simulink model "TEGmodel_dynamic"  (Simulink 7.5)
settings: Solver=ode23s  StartTime=0.0  StopTime=0.01  RelTol=1e-3
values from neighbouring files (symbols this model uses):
  alpha = 0.000382    [TEGmodel_contactR.m]    (also in TEGmodel_parameters.m; TEGmodel_simplified.m)
  mtcs = 0.4492*7.7/1000    (= 0.00345884)    [TEGmodel_parameters.m]
  N = 72    [TEGmodel_contactR.m]    (also in TEGmodel_parameters.m; TEGmodel_simplified.m)
  Ri = 10.2    [TEGmodel_parameters.m]    (also in TEGmodel_simplified.m)
  RL = 10.2    [TEGmodel_parameters.m]    (also in TEGmodel_simplified.m)
  TC = 35 + CtoK    (= 308.15)    [TEGmodel_contactR.m]    (also in TEGmodel_parameters.m; TEGmodel_simplified.m = 35)
  TH = 85 + CtoK    (= 358.15)    [TEGmodel_contactR.m]    (also in TEGmodel_parameters.m; TEGmodel_simplified.m = 85)
libraries: fl_lib x30, nesl_utility x13

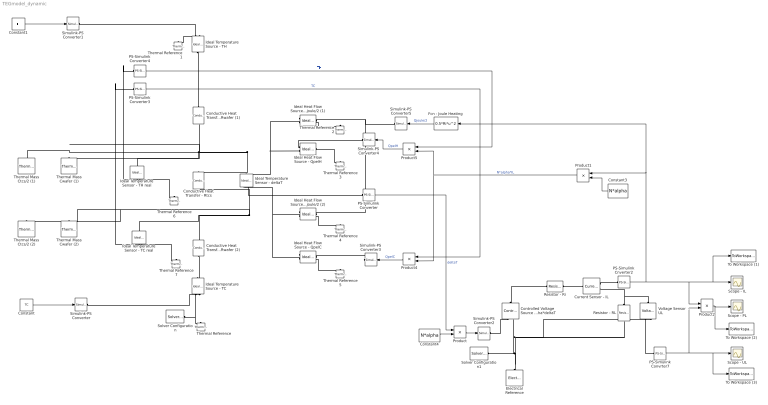
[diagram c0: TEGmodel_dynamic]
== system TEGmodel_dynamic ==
  Conductive Heat Transfer - Rtcs : fl_lib/Thermal/Thermal Elements/Conductive Heat Transfer  DialogController=NetworkEngine.DynNeDlgSource  SystemSampleTime=-1  area=Atcs mm^2  thickness=ttcs mm  th_cond=ktcs W/(m*K)  Q_Log=off  T_Log=off  LocalVarNames=|Q|T  LocalVarDescs=|Q|T  LocalVarLogging=[0 0]
  Conductive Heat Transfer - Rwafer (1) : fl_lib/Thermal/Thermal Elements/Conductive Heat Transfer  DialogController=NetworkEngine.DynNeDlgSource  SystemSampleTime=-1  area=Awafer mm^2  thickness=twafer mm  th_cond=kwafer W/(m*K)  Q_Log=off  T_Log=off  LocalVarNames=|Q|T  LocalVarDescs=|Q|T  LocalVarLogging=[0 0]
  Conductive Heat Transfer - Rwafer (2) : fl_lib/Thermal/Thermal Elements/Conductive Heat Transfer  DialogController=NetworkEngine.DynNeDlgSource  SystemSampleTime=-1  area=Awafer mm^2  thickness=twafer mm  th_cond=kwafer W/(m*K)  Q_Log=off  T_Log=off  LocalVarNames=|Q|T  LocalVarDescs=|Q|T  LocalVarLogging=[0 0]
  Constant : Constant  Value=TC  OutDataType=fixdt(1, 16)  OutScaling=2^0
  Constant1 : Constant  Value=TH  OutDataType=fixdt(1, 16)  OutScaling=2^0
  Constant3 : Constant  Value=N*alpha  OutDataType=fixdt(1, 16)  OutScaling=2^0
  Constant4 : Constant  Value=N*alpha  OutDataType=fixdt(1, 16)  OutScaling=2^0
  Controlled Voltage Source  - N*alpha*deltaT : fl_lib/Electrical/Electrical Sources/Controlled Voltage Source  DialogController=NetworkEngine.DynNeDlgSource  SystemSampleTime=-1  i_Log=off  v_Log=off  LocalVarNames=|i|v  LocalVarDescs=|i|v  LocalVarLogging=[0 0]
  Current Sensor - IL : fl_lib/Electrical/Electrical Sensors/Current Sensor  DialogController=NetworkEngine.DynNeDlgSource  SystemSampleTime=-1  i1_Log=off  v1_Log=off  LocalVarNames=|i1|v1  LocalVarDescs=|i1|v1  LocalVarLogging=[0 0]
  Electrical Reference : fl_lib/Electrical/Electrical Elements/Electrical Reference  DialogController=NetworkEngine.DynNeDlgSource  SystemSampleTime=-1  i_Log=off  LocalVarNames=|i  LocalVarDescs=|i  LocalVarLogging=0
  Fcn - Joule Heating : Fcn  Expr=0.5*Ri*u^2
  Ideal Heat Flow Source - Qjoule/2 (1) : fl_lib/Thermal/Thermal Sources/Ideal Heat Flow Source  DialogController=NetworkEngine.DynNeDlgSource  SystemSampleTime=-1  Q_Log=off  T_Log=off  LocalVarNames=|Q|T  LocalVarDescs=|Q|T  LocalVarLogging=[0 0]
  Ideal Heat Flow Source - Qjoule/2 (2) : fl_lib/Thermal/Thermal Sources/Ideal Heat Flow Source  DialogController=NetworkEngine.DynNeDlgSource  SystemSampleTime=-1  Q_Log=off  T_Log=off  LocalVarNames=|Q|T  LocalVarDescs=|Q|T  LocalVarLogging=[0 0]
  Ideal Heat Flow Source - QpelC : fl_lib/Thermal/Thermal Sources/Ideal Heat Flow Source  DialogController=NetworkEngine.DynNeDlgSource  SystemSampleTime=-1  Q_Log=off  T_Log=off  LocalVarNames=|Q|T  LocalVarDescs=|Q|T  LocalVarLogging=[0 0]
  Ideal Heat Flow Source - QpelH : fl_lib/Thermal/Thermal Sources/Ideal Heat Flow Source  DialogController=NetworkEngine.DynNeDlgSource  SystemSampleTime=-1  Q_Log=off  T_Log=off  LocalVarNames=|Q|T  LocalVarDescs=|Q|T  LocalVarLogging=[0 0]
  Ideal Temperature Sensor - TC real : fl_lib/Thermal/Thermal Sensors/Ideal Temperature Sensor  DialogController=NetworkEngine.DynNeDlgSource  SystemSampleTime=-1  Qs_Log=off  Ts_Log=off  LocalVarNames=|Qs|Ts  LocalVarDescs=|Qs|Ts  LocalVarLogging=[0 0]
  Ideal Temperature Sensor - TH real : fl_lib/Thermal/Thermal Sensors/Ideal Temperature Sensor  DialogController=NetworkEngine.DynNeDlgSource  SystemSampleTime=-1  Qs_Log=off  Ts_Log=off  LocalVarNames=|Qs|Ts  LocalVarDescs=|Qs|Ts  LocalVarLogging=[0 0]
  Ideal Temperature Sensor - deltaT : fl_lib/Thermal/Thermal Sensors/Ideal Temperature Sensor  DialogController=NetworkEngine.DynNeDlgSource  SystemSampleTime=-1  Qs_Log=off  Ts_Log=off  LocalVarNames=|Qs|Ts  LocalVarDescs=|Qs|Ts  LocalVarLogging=[0 0]
  Ideal Temperature Source - TC : fl_lib/Thermal/Thermal Sources/Ideal Temperature Source  DialogController=NetworkEngine.DynNeDlgSource  SystemSampleTime=-1  Q_Log=off  T_Log=off  LocalVarNames=|Q|T  LocalVarDescs=|Q|T  LocalVarLogging=[0 0]
  Ideal Temperature Source - TH : fl_lib/Thermal/Thermal Sources/Ideal Temperature Source  DialogController=NetworkEngine.DynNeDlgSource  SystemSampleTime=-1  Q_Log=off  T_Log=off  LocalVarNames=|Q|T  LocalVarDescs=|Q|T  LocalVarLogging=[0 0]
  PS-Simulink Cnverter2 : nesl_utility/PS-Simulink Converter  DialogController=NetworkEngine.DynNeUtilDlgSource  SystemSampleTime=-1  PhysicalDomain=network_engine_domain  LeftPortType=input  RightPortType=output  SubClassName=ps_output  Unit=1  AffineConversion=off
  PS-Simulink Converter : nesl_utility/PS-Simulink Converter  DialogController=NetworkEngine.DynNeUtilDlgSource  SystemSampleTime=-1  PhysicalDomain=network_engine_domain  LeftPortType=input  RightPortType=output  SubClassName=ps_output  Unit=1  AffineConversion=off
  PS-Simulink Converter3 : nesl_utility/PS-Simulink Converter  DialogController=NetworkEngine.DynNeUtilDlgSource  SystemSampleTime=-1  PhysicalDomain=network_engine_domain  LeftPortType=input  RightPortType=output  SubClassName=ps_output  Unit=1  AffineConversion=off
  PS-Simulink Converter4 : nesl_utility/PS-Simulink Converter  DialogController=NetworkEngine.DynNeUtilDlgSource  SystemSampleTime=-1  PhysicalDomain=network_engine_domain  LeftPortType=input  RightPortType=output  SubClassName=ps_output  Unit=1  AffineConversion=off
  PS-Simulink Convrter7 : nesl_utility/PS-Simulink Converter  DialogController=NetworkEngine.DynNeUtilDlgSource  SystemSampleTime=-1  PhysicalDomain=network_engine_domain  LeftPortType=input  RightPortType=output  SubClassName=ps_output  Unit=1  AffineConversion=off
  Product{,1..2,4..5} (5 alike) : Product  OutDataType=fixdt(1, 16)  OutScaling=2^0
  Resistor - RL : fl_lib/Electrical/Electrical Elements/Resistor  DialogController=NetworkEngine.DynNeDlgSource  SystemSampleTime=-1  R=RL Ohm  i_Log=off  v_Log=off  LocalVarNames=|i|v  LocalVarDescs=|i|v  LocalVarLogging=[0 0]
  Resistor - Ri : fl_lib/Electrical/Electrical Elements/Resistor  DialogController=NetworkEngine.DynNeDlgSource  SystemSampleTime=-1  R=Ri Ohm  i_Log=off  v_Log=off  LocalVarNames=|i|v  LocalVarDescs=|i|v  LocalVarLogging=[0 0]
  Scope - IL : Scope
  Scope - PL : Scope
  Scope - UL : Scope
  Simulink-PS Converter{,1..5} (6 alike) : nesl_utility/Simulink-PS Converter  DialogController=NetworkEngine.DynNeUtilDlgSource  SystemSampleTime=-1  PhysicalDomain=network_engine_domain  LeftPortType=input  RightPortType=output  SubClassName=ps_input  Unit=1  AffineConversion=off  InputFilterTimeConstant=.001  UdotUserProvided=0
  Solver Configuration : nesl_utility/Solver Configuration  DialogController=NetworkEngine.DynNeUtilDlgSource  SystemSampleTime=-1  PhysicalDomain=network_engine_domain  LeftPortType=input  RightPortType=generic  SubClassName=solver  Accelerate=off  Profile=off  ResidualTolerance=1e-9  MaxNonlinIter=3  MaxModeIter=2  DoFixedCost=off  UseLocalSampling=off  DoDC=off  LinearAlgebra=Sparse  LocalSolverSampleTime=.001  LocalSolverChoice=NE_BACKWARD_EULER_ADVANCER  UseLocalSolver=off
  Solver Configuration1 : nesl_utility/Solver Configuration  DialogController=NetworkEngine.DynNeUtilDlgSource  SystemSampleTime=-1  PhysicalDomain=network_engine_domain  LeftPortType=input  RightPortType=generic  SubClassName=solver  Accelerate=off  Profile=off  ResidualTolerance=1e-9  MaxNonlinIter=3  MaxModeIter=2  DoFixedCost=off  UseLocalSampling=off  DoDC=off  LinearAlgebra=Sparse  LocalSolverSampleTime=.001  LocalSolverChoice=NE_BACKWARD_EULER_ADVANCER  UseLocalSolver=off
  Thermal Mass Ctcs/2 (1) : fl_lib/Thermal/Thermal Elements/Thermal Mass  DialogController=NetworkEngine.DynNeDlgSource  SystemSampleTime=-1  mass=mtcs/2 g  sp_heat=Cspecwafer J/kg/K  init_temp=TC K  Q_Log=off  LocalVarNames=|Q  LocalVarDescs=|Q  LocalVarLogging=0
  Thermal Mass Ctcs/2 (2) : fl_lib/Thermal/Thermal Elements/Thermal Mass  DialogController=NetworkEngine.DynNeDlgSource  SystemSampleTime=-1  mass=mtcs/2 g  sp_heat=Cspectcs J/kg/K  init_temp=TC K  Q_Log=off  LocalVarNames=|Q  LocalVarDescs=|Q  LocalVarLogging=0
  Thermal Mass Cwafer (1) : fl_lib/Thermal/Thermal Elements/Thermal Mass  DialogController=NetworkEngine.DynNeDlgSource  SystemSampleTime=-1  mass=mwafer g  sp_heat=Cspecwafer J/kg/K  init_temp=TC K  Q_Log=off  LocalVarNames=|Q  LocalVarDescs=|Q  LocalVarLogging=0
  Thermal Mass Cwafer (2) : fl_lib/Thermal/Thermal Elements/Thermal Mass  DialogController=NetworkEngine.DynNeDlgSource  SystemSampleTime=-1  mass=mwafer g  sp_heat=Cspecwafer J/kg/K  init_temp=TC K  Q_Log=off  LocalVarNames=|Q  LocalVarDescs=|Q  LocalVarLogging=0
  Thermal Reference{,1..7} (8 alike) : fl_lib/Thermal/Thermal Elements/Thermal Reference  DialogController=NetworkEngine.DynNeDlgSource  SystemSampleTime=-1  Q_Log=off  LocalVarNames=|Q  LocalVarDescs=|Q  LocalVarLogging=0
  To Workspace (1) : ToWorkspace  VariableName=IL  SampleTime=-1  SaveFormat=Array
  To Workspace (2) : ToWorkspace  VariableName=PL  SampleTime=-1  SaveFormat=Array
  To Workspace (3) : ToWorkspace  VariableName=UL  SampleTime=-1  SaveFormat=Array
  Voltage Sensor  - UL : fl_lib/Electrical/Electrical Sensors/Voltage Sensor  DialogController=NetworkEngine.DynNeDlgSource  SystemSampleTime=-1  i1_Log=off  v1_Log=off  LocalVarNames=|i1|v1  LocalVarDescs=|i1|v1  LocalVarLogging=[0 0]
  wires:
  Constant/1 -> Simulink-PS Converter/1
  Constant1/1 -> Simulink-PS Converter1/1
  Product/1 -> Simulink-PS Converter2/1
  PS-Simulink Cnverter2/1 -> Product2/1, Scope - IL/1, To Workspace (1)/1, Fcn - Joule Heating/1, Product1/1
  PS-Simulink Convrter7/1 -> Product2/2, Scope - UL/1, To Workspace (3)/1
  Fcn - Joule Heating/1 -> Simulink-PS Converter5/1  "Qjoule/2"
  PS-Simulink Converter/1 -> Product/1  "deltaT"
  Constant4/1 -> Product/2
  PS-Simulink Converter3/1 -> Product4/1  "TC"
  Product4/1 -> Simulink-PS Converter3/1  "QpelC"
  Product5/1 -> Simulink-PS Converter4/1  "QpelH"
  PS-Simulink Converter4/1 -> Product5/1  "TH"
  Product2/1 -> Scope - PL/1, To Workspace (2)/1
  Product1/1 -> Product5/2, Product4/2  "N*alpha*IL"
  Constant3/1 -> Product1/2
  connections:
  Solver Configuration/RConn1 -- Thermal Reference/LConn1 -- Ideal Temperature Source - TC/RConn2
  Ideal Heat Flow Source - Qjoule/2 (1)/LConn1 -- Conductive Heat Transfer - Rtcs/RConn1 -- Ideal Temperature Sensor - TH real/LConn1 -- Conductive Heat Transfer - Rwafer (1)/LConn1 -- Thermal Mass Ctcs/2 (1)/LConn1 -- Thermal Mass Cwafer (1)/LConn1 -- Ideal Heat Flow Source - QpelH/RConn2 -- Ideal Temperature Sensor - deltaT/LConn1
  Ideal Heat Flow Source - QpelH/LConn1 -- Thermal Reference3/LConn1
  Ideal Heat Flow Source - Qjoule/2 (1)/RConn2 -- Thermal Reference2/LConn1
  Ideal Heat Flow Source - Qjoule/2 (2)/RConn2 -- Thermal Reference4/LConn1
  Ideal Heat Flow Source - QpelC/RConn2 -- Thermal Reference5/LConn1
  Ideal Heat Flow Source - QpelC/LConn1 -- Ideal Heat Flow Source - Qjoule/2 (2)/LConn1 -- Conductive Heat Transfer - Rtcs/LConn1 -- Ideal Temperature Sensor - TC real/LConn1 -- Conductive Heat Transfer - Rwafer (2)/RConn1 -- Thermal Mass Cwafer (2)/LConn1 -- Thermal Mass Ctcs/2 (2)/LConn1 -- Ideal Temperature Sensor - deltaT/RConn1
  Simulink-PS Converter/RConn1 -- Ideal Temperature Source - TC/RConn1
  Electrical Reference/LConn1 -- Controlled Voltage Source  - N*alpha*deltaT/RConn2 -- Resistor - RL/RConn1 -- Voltage Sensor  - UL/RConn2 -- Solver Configuration1/RConn1
  Controlled Voltage Source  - N*alpha*deltaT/LConn1 -- Resistor - Ri/LConn1
  Resistor - RL/LConn1 -- Current Sensor - IL/RConn2 -- Voltage Sensor  - UL/LConn1
  Simulink-PS Converter2/RConn1 -- Controlled Voltage Source  - N*alpha*deltaT/RConn1
  Resistor - Ri/RConn1 -- Current Sensor - IL/LConn1
  Current Sensor - IL/RConn1 -- PS-Simulink Cnverter2/LConn1
  Ideal Temperature Sensor - TH real/RConn1 -- Thermal Reference6/LConn1
  Ideal Temperature Sensor - TC real/RConn1 -- Thermal Reference7/LConn1
  Ideal Temperature Sensor - TH real/RConn2 -- PS-Simulink Converter4/LConn1
  Ideal Temperature Sensor - TC real/RConn2 -- PS-Simulink Converter3/LConn1
  Simulink-PS Converter3/RConn1 -- Ideal Heat Flow Source - QpelC/RConn1
  Ideal Heat Flow Source - QpelH/RConn1 -- Simulink-PS Converter4/RConn1
  Voltage Sensor  - UL/RConn1 -- PS-Simulink Convrter7/LConn1
  Ideal Heat Flow Source - Qjoule/2 (2)/RConn1 -- Ideal Heat Flow Source - Qjoule/2 (1)/RConn1 -- Simulink-PS Converter5/RConn1
  Ideal Temperature Source - TH/LConn1 -- Conductive Heat Transfer - Rwafer (1)/RConn1
  Ideal Temperature Source - TH/RConn2 -- Thermal Reference1/LConn1
  Ideal Temperature Sensor - deltaT/RConn2 -- PS-Simulink Converter/LConn1
  Simulink-PS Converter1/RConn1 -- Ideal Temperature Source - TH/RConn1
  Conductive Heat Transfer - Rwafer (2)/LConn1 -- Ideal Temperature Source - TC/LConn1
